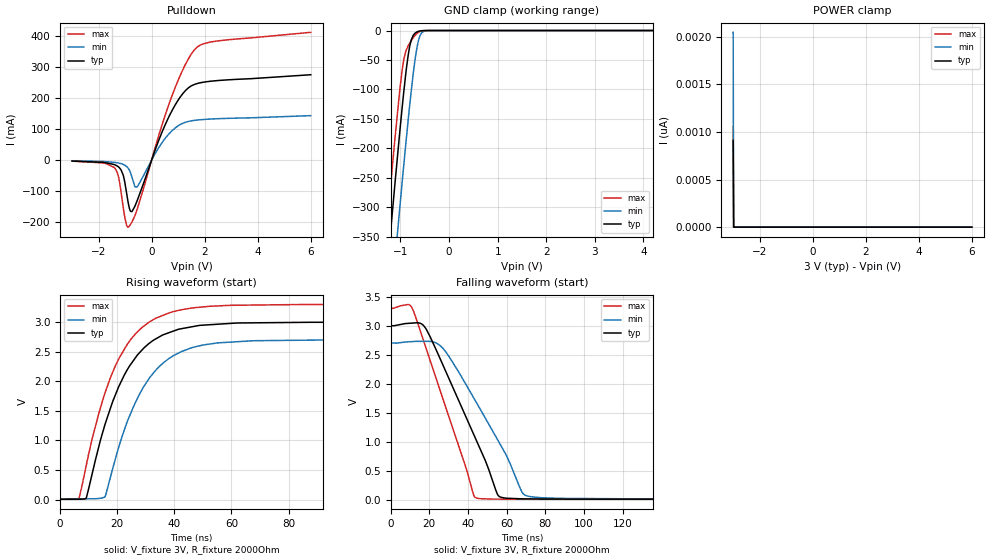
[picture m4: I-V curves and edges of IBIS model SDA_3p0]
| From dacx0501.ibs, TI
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|   Model
[Model]   SDA_3p0
Model_type   I/O_open_drain
Polarity   Non-Inverting
Enable   Active-Low
Vinl = 0.9
Vinh = 2.1
Vmeas = 1.5
Vref = 3
Cref = 1pF
Rref = 2000
|   typ   min   max
C_comp   3.377pF   3.057pF   3.504pF
[Voltage Range]   3   2.7   3.3
[Temperature Range]   25   125   -40
[Pullup Reference]   3   2.7   3.3
[Pulldown Reference]   0   0   0
[Power Clamp Reference]   3   2.7   3.3
[GND Clamp Reference]   0   0   0
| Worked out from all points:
|   slope of the pulldown table from 0 to 0.45 V, typ, clamps not added: 4.43 ohm
|   GND clamp passes 1 mA (typ) near -0.61 V on its own axis
|   falling waveform, V_fixture 3V, R_fixture 2000Ohm: 20-80 % time 23.8ns typ, 26.9ns min, 19.8ns max; typ from 3 V to 0.006 V
|   rising waveform, V_fixture 3V, R_fixture 2000Ohm: 20-80 % time 14.4ns typ, 14.5ns min, 14.2ns max; typ from 0.006 V to 3 V
[Pulldown]
|   Voltage   I(typ)   I(min)   I(max)
-3V       -3.218mA   -2.249mA   -3.536mA
-1.389V   -15.19mA   -7.59mA    -25.7mA
-1.245V   -22.47mA   -9.606mA   -55.36mA
-1.074V   -48.2mA    -13.93mA   -150.9mA
-948mV    -104.3mA   -20.47mA   -209.2mA
-876mV    -140.8mA   -27.35mA   -215.7mA
-741mV    -165.9mA   -55.54mA   -199.4mA
-552mV    -132.1mA   -86.56mA   -160.3mA
663mV     141.6mA    85.19mA    182.4mA
1.158V    212.1mA    117.9mA    287.6mA
1.653V    244.8mA    128.2mA    358.9mA
6V        274.8mA    143mA      411.5mA
[GND Clamp]
|   Voltage   I(typ)   I(min)   I(max)
-3V       -2.092A    -2.219A    -2.017A
-1.353V   -483.7mA   -616.1mA   -404.6mA
-1.182V   -323.5mA   -455.6mA   -245.3mA
-1.119V   -265.8mA   -397.3mA   -188.9mA
-1.011V   -170.2mA   -299.1mA   -99.41mA
-930mV    -103.4mA   -227.6mA   -49.25mA
-840mV    -41.78mA   -151.7mA   -25.95mA
-777mV    -15.92mA   -102.4mA   -17.11mA
-651mV    -2.067mA   -25.52mA   -4.429mA
-570mV    -384.2uA   -4.886mA   -894.8uA
-426mV    -8.62uA    -122uA     -11.74uA
6V        0A         0A         0A
[POWER Clamp]
|   Voltage   I(typ)   I(min)   I(max)
-3V       912.4pA    2.049nA    1.062nA
-2.982V   0A         0A         0A
-2.973V   0A         0A         0A
6V        0A         0A         0A
[Ramp]
R_load = 2000
|   typ   min   max
dV/dt_r   1.79642/1.43273e-08   1.61502/1.44667e-08   1.97679/1.42031e-08
dV/dt_f   1.79642/2.38051e-08   1.61502/2.68781e-08   1.97679/1.98311e-08
[Falling Waveform]
V_fixture = 3V
V_fixture_min = 2.7V
V_fixture_max = 3.3V
R_fixture = 2000Ohm
C_fixture = 0F
|   Time   V(typ)   V(min)   V(max)
0s        3V         2.7V       3.3V
11.35ns   3.043V     2.725V     3.284V
17.92ns   2.961V     2.728V     2.647V
26.84ns   2.334V     2.614V     1.754V
42.93ns   1.125V     1.754V     79.64mV
45.03ns   967.7mV    1.634V     21.77mV
55.63ns   70.04mV    1.012V     8.883mV
67.9ns    14.33mV    130.7mV    7.349mV
72.84ns   12.36mV    48.8mV     6.73mV
500ns     5.964mV    8.292mV    5.357mV
[Rising Waveform]
V_fixture = 3V
V_fixture_min = 2.7V
V_fixture_max = 3.3V
R_fixture = 2000Ohm
C_fixture = 0F
|   Time   V(typ)   V(min)   V(max)
0s        5.964mV    8.29mV     5.357mV
6.583ns   7.73mV     12.12mV    16.46mV
9.217ns   38.49mV    13.65mV    594.8mV
15.61ns   1.254V     45.33mV    1.789V
23.54ns   2.199V     1.323V     2.63V
27.43ns   2.465V     1.75V      2.853V
33.26ns   2.712V     2.176V     3.061V
45.98ns   2.922V     2.567V     3.24V
90.92ns   2.999V     2.699V     3.3V
500ns     3V         2.7V       3.3V
